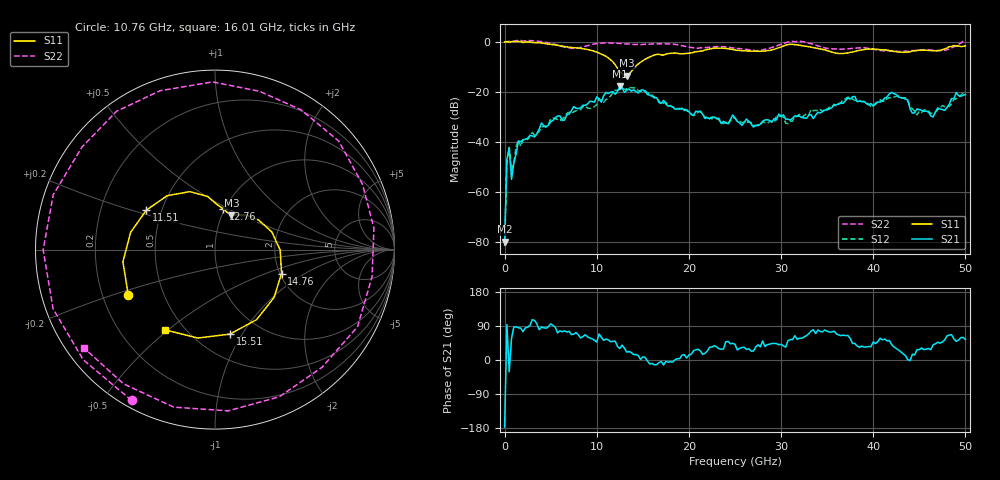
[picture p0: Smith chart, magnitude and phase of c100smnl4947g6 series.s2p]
! 3/5/2025 12:34:24 PM
! D:\C100SMNL4947G6 SERIES.S2P
! CHANNEL.1
! TR.MEASUREMENT
! CORRECTED.DATA
# GHZ S RI R 50.0
! FREQ.GHZ  S11RE  S11IM  S21RE  S21IM  S12RE  S12IM  S22RE  S22IM
!; PortSelection: Port_12
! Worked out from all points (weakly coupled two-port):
!   201 points, 10 MHz to 50 GHz, reference 50 ohm
!   highest |S21| = -17.61 dB at 12.51 GHz (marker M1); lowest = -79.9 dB at 10 MHz (marker M2)
!   lowest |S11| = -13.5 dB at 13.26 GHz (marker M3), VSWR 1.53, Z = 55.4 + j22.1 ohm
!   |S11| at or under -10 dB: 12.17 GHz to 14.16 GHz (1.986 GHz wide, 15.1 % of centre)
!   |S22| runs from -3.8 to 0.6 dB; largest |S21 - S12| = 0.041
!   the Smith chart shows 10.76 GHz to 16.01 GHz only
!   S11 on the Smith chart (normalised r, x): 10.76 GHz: 0.31, -0.22; 11.51 GHz: 0.41, +0.22; 12.76 GHz: 0.98, +0.47; 14.76 GHz: 2.04, -0.64; 15.51 GHz: 0.73, -0.89; 16.01 GHz: 0.39, -0.49
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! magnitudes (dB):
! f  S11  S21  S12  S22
! 10 MHz  0.0  -79.9  -81.7  0.1
! 259.9 MHz  0.2  -46.9  -48.1  0.2
! 509.9 MHz  -0.1  -42.3  -42.1  0.3
! 759.9 MHz  0.2  -54.9  -51.2  0.3
! 1.51 GHz  0.2  -39.7  -39.1  0.6
! 8.508 GHz  -2.7  -25.3  -25.9  -1.9
! 10.76 GHz  -5.3  -21.5  -24.1  -0.4
! 11.51 GHz  -7.1  -20.1  -21.6  -0.4
! 12.51 GHz  -12.0  -17.6  -18.8  -0.6
! 12.76 GHz  -12.7  -18.3  -18.5  -0.6
! 13.26 GHz  -13.5  -19.3  -18.8  -0.8
! 14.76 GHz  -8.1  -19.3  -19.8  -1.0
! 15.51 GHz  -6.4  -21.0  -20.2  -0.8
! 16.01 GHz  -5.6  -21.7  -21.2  -0.8
! 16.76 GHz  -4.9  -24.2  -23.6  -0.7
! 25 GHz  -3.2  -30.3  -30.6  -2.6
! 30.75 GHz  -1.0  -30.9  -32.7  0.0
! 33.5 GHz  -2.2  -30.6  -27.5  -0.9
! 37.25 GHz  -4.4  -22.4  -22.1  -2.7
! 41.75 GHz  -3.5  -20.8  -22.3  -3.6
! 46.5 GHz  -3.5  -30.0  -28.6  -3.2
! 50 GHz  -1.5  -21.0  -21.0  0.5
